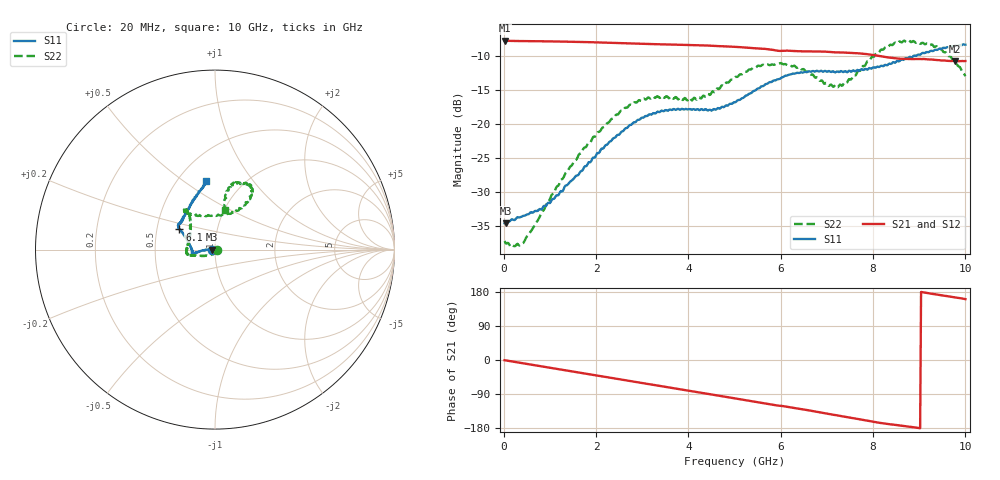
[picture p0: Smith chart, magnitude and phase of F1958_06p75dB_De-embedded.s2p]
! Integrated Device Technology
! Corporate Headquarters
! 6024 Silver Creek Valley Road
! San Jose, CA 95138  USA
! Phone:  1-408-284-8200
! Toll Free:  1-800-223-1366
! Webpage:  http://www.idt.com/
! Timing and RF Division
! 515 Groton Road, Suite 102
! Westford, MA 01886-6024
! Device:  F1958
! Description: 7-bit 0.25 dB Digital Step Attenuator
! Frequency:  0.001 -  6.000 GHz
! Package:  4x4 mm Thin QFN Plastic Package: 24 pin
! Ports:  2 RF, 12 DC
!  Pin  1  = D0
!  Pin  2  = VDD
!  Pin  3  = VMODE
!  Pin  4  = GND
!  Pin  5  = RF1  =  Port 1
!  Pin  6  = GND
!  Pin  7  = GND
!  Pin  8  = GND
!  Pin  9  = GND
!  Pin 10  = GND
!  Pin 11  = GND
!  Pin 12  = GND
!  Pin 13  = GND
!  Pin 14  = RF2  =  Port 2
!  Pin 15  = GND
!  Pin 16  = LE
!  Pin 17  = CLK
!  Pin 18  = DATA
!  Pin 19  = D6
!  Pin 20  = D5
!  Pin 21  = D4
!  Pin 22  = D3
!  Pin 23  = D2
!  Pin 24  = D1
! State:  27
! Atten State:  6.75 dB
! Voltage:  +3.30 Volts
! Current:  0.257 mA
! Data:  The device was measured on a F1958 evaluation board which has
!  individual transmission lines to the RF pins.  Data was collected
!  using a calibrated network analyzer.  The evaluation board was
!  de-embedded using Automatic Fixture Removal (AFR).
!  The reference plane is the edge of the package pin.
! Misc:
!  Action Tracker AT0419
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# GHz S dB R 50
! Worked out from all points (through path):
!   500 points, 20 MHz to 10 GHz, reference 50 ohm
!   highest |S21| = -7.69 dB at 20 MHz (marker M1); lowest = -10.7 dB at 9.78 GHz (marker M2)
!   group delay of S21, straight-line fit = 55.7 ps
!   lowest |S11| = -34.6 dB at 40 MHz (marker M3), VSWR 1.04, Z = 48.2 - j0.0872 ohm
!   |S11| at or under -10 dB: start of sweep to 8.867 GHz
!   |S22| runs from -37.9 to -7.7 dB; largest |S21 - S12| = 0.0012
!   S11 on the Smith chart (normalised r, x): 20 MHz: 0.96, -0.00; 6.1 GHz: 0.65, +0.15; 10 GHz: 0.68, +0.61
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0.02  -34.53 -177.5  -7.69 -0.6  -7.69 -0.5  -37.15 -10.4
0.04  -34.56 -177.2  -7.70 -1.0  -7.70 -0.9  -37.44 -16.0
0.2  -34.00 178.9  -7.73 -4.2  -7.73 -4.2  -37.81 -36.2
0.42  -33.45 174.9  -7.75 -8.7  -7.75 -8.6  -37.46 -62.2
0.96  -31.53 177.1  -7.79 -19.6  -7.79 -19.6  -31.40 -110.6
1.7  -26.82 -177.6  -7.89 -34.5  -7.88 -34.5  -23.97 -147.7
2.58  -21.01 -172.0  -8.06 -52.3  -8.04 -52.3  -17.97 -164.8
3.36  -18.18 -168.8  -8.22 -68.0  -8.22 -68.1  -16.03 -173.3
4.22  -17.83 -172.2  -8.37 -85.3  -8.38 -85.4  -16.00 156.5
4.54  -17.76 -178.8  -8.47 -91.8  -8.48 -91.9  -15.18 143.8
5.02  -16.73 167.7  -8.60 -101.6  -8.61 -101.6  -13.01 129.1
5.52  -14.70 156.6  -8.84 -111.7  -8.85 -111.7  -11.36 125.9
6.1  -12.84 150.6  -9.17 -122.7  -9.18 -122.7  -11.13 127.9
6.68  -12.19 146.4  -9.27 -134.3  -9.29 -134.3  -12.66 122.0
7.04  -12.15 143.2  -9.33 -142.4  -9.35 -142.3  -14.32 104.9
7.3  -12.16 141.2  -9.42 -147.7  -9.42 -147.6  -14.17 84.6
7.9  -11.82 130.3  -9.70 -160.8  -9.69 -160.8  -10.69 57.9
8.34  -11.11 120.7  -10.17 -169.2  -10.17 -169.3  -8.52 56.4
8.74  -10.34 112.4  -10.39 -175.1  -10.40 -175.1  -7.82 61.7
9.24  -9.21 102.7  -10.46 175.3  -10.47 175.3  -8.34 72.7
9.78  -8.42 98.1  -10.71 165.2  -10.73 165.3  -10.70 78.4
10  -8.28 97.9  -10.68 160.6  -10.72 160.7  -12.92 75.5
